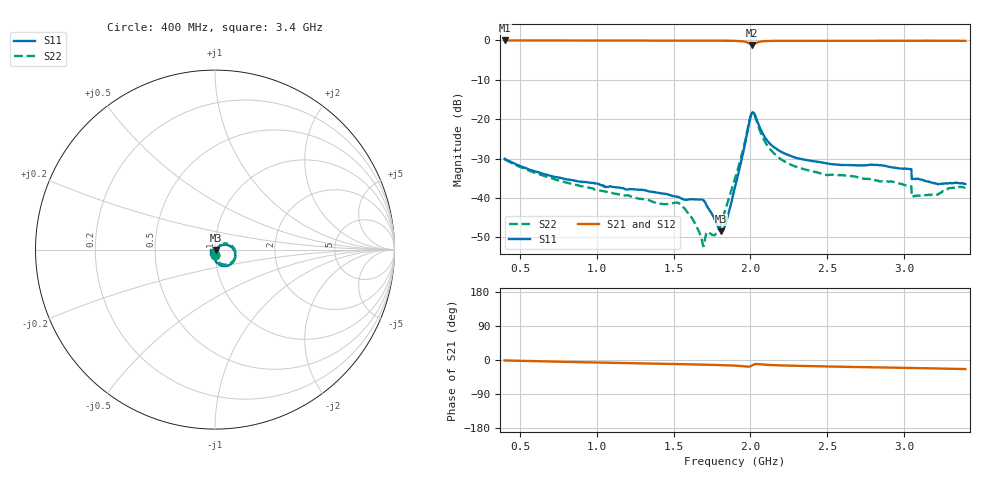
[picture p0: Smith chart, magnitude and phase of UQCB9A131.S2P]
!  Part Number  UQCB9A131	Mounting Orientation: Vertical
!  Description: RF capacitors
!  Application: Coupling, Bypass, Tuning, DC Block
!  Filters, Matching
# GHZ S DB R 50
! Freq  |S11|  S11 Ph  |S21|  S21 Ph  |S12|  S12 Ph  |S22|  S22 Ph
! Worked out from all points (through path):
!   801 points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, 400 MHz to 3.4 GHz, reference 50 ohm
!   highest |S21| = -0.02 dB at 400 MHz (marker M1); lowest = -1.2 dB at 2.013 GHz (marker M2)
!   group delay of S21, straight-line fit = 19.8 ps
!   lowest |S11| = -48.4 dB at 1.81 GHz (marker M3), VSWR 1.01, Z = 50.3 - j0.216 ohm
!   |S11| at or under -10 dB: start of sweep to end of sweep
!   |S22| runs from -52.2 to -18.4 dB; largest |S21 - S12| = 0.0024
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0.4  -30.04 -88.4  -0.02 -1.2  -0.01 -1.2  -30.16 -88.3
0.651  -33.87 -87.5  -0.03 -3.7  -0.01 -3.7  -34.32 -87.7
0.903  -35.86 -86.9  -0.03 -5.8  -0.02 -5.8  -37.00 -87.1
1.401  -38.72 -87.1  -0.05 -9.8  -0.03 -9.8  -41.39 -80.7
1.548  -40.04 -84.9  -0.06 -11.0  -0.05 -11.0  -41.69 -85.4
1.623  -40.32 -77.8  -0.06 -11.6  -0.04 -11.7  -45.25 -86.3
1.69  -40.47 -80.0  -0.07 -12.3  -0.06 -12.3  -51.78 -58.0
1.724  -42.46 -82.4  -0.07 -12.5  -0.06 -12.6  -48.60 -30.8
1.773  -45.85 -69.4  -0.08 -13.0  -0.06 -13.1  -49.21 -3.0
1.81  -48.43 -34.4  -0.08 -13.4  -0.07 -13.5  -46.33 28.4
1.848  -45.34 10.6  -0.09 -13.9  -0.08 -13.9  -41.63 44.0
1.9  -37.10 37.6  -0.12 -14.8  -0.11 -14.8  -34.99 50.1
1.99  -21.30 12.9  -0.73 -17.5  -0.71 -17.5  -21.09 18.3
2.013  -18.30 -23.6  -1.17 -14.0  -1.16 -14.0  -18.42 -19.1
2.091  -24.42 -88.8  -0.20 -12.3  -0.19 -12.3  -25.45 -85.3
2.151  -27.02 -96.2  -0.13 -13.6  -0.11 -13.6  -28.60 -92.6
2.256  -29.22 -101.5  -0.10 -14.9  -0.09 -15.0  -31.41 -96.7
2.403  -30.60 -104.7  -0.10 -16.3  -0.09 -16.3  -33.20 -99.3
2.901  -32.07 -112.8  -0.12 -19.9  -0.11 -20.0  -35.89 -104.7
3.033  -32.67 -113.9  -0.11 -20.9  -0.09 -20.9  -36.91 -109.4
3.066  -35.13 -115.4  -0.10 -21.1  -0.09 -21.1  -39.46 -80.5
3.4  -36.45 -125.5  -0.11 -23.9  -0.10 -24.0  -37.35 -81.5
